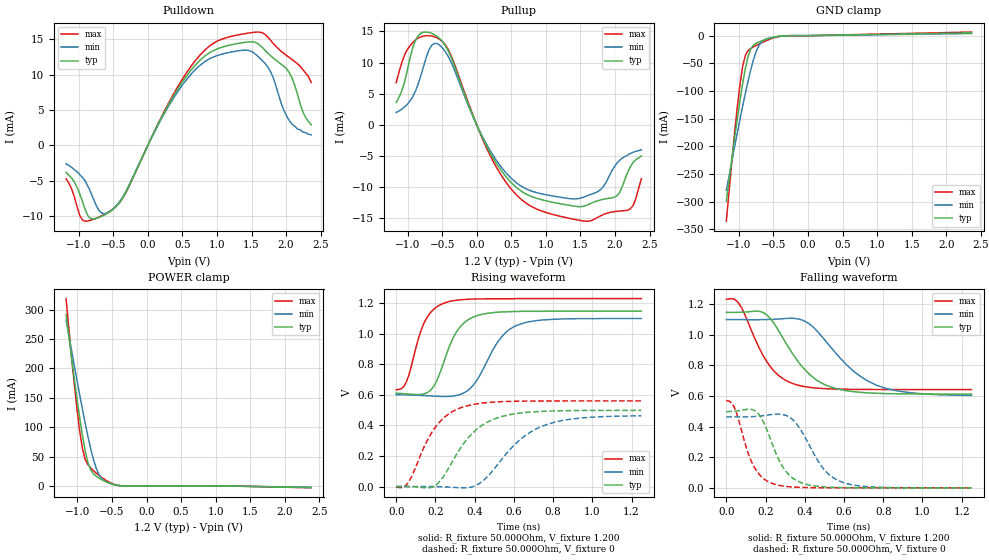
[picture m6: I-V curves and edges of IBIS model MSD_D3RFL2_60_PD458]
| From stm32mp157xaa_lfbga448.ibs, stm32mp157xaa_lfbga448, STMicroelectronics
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[Model] MSD_D3RFL2_60_PD458
Model_type   I/O
C_comp 2.402pF   2.316pF   2.526pF
Vinh = 820.000mV
Vinl = 380.000mV
Vmeas = 600.000mV
Vref = 600.000mV
[Model Spec]
Vinh   820.000mV   790.000mV   870.000mV
Vinl   380.000mV   350.000mV   430.000mV
Vmeas   600.000mV   570.000mV   650.000mV
Vref   600.000mV   570.000mV   650.000mV
[Temperature Range]   25.000   125.000   -40.000
[Voltage Range]   1.200V   1.140V   1.300V
[GND Clamp Reference]   0.00V   0.00V   0.00V
[Pulldown Reference]   0.00V   0.00V   0.00V
[POWER Clamp Reference]   1.200V   1.140V   1.300V
[Pullup Reference]   1.200V   1.140V   1.300V
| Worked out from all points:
|   slope of the pulldown table from 0 to 0.18 V, typ, clamps not added: 50.1 ohm
|   slope of the pullup table from 0 to 0.18 V, typ, clamps not added: 42.9 ohm
|   GND clamp passes 1 mA (typ) near -0.40 V on its own axis
|   POWER clamp passes 1 mA (typ) near -0.41 V on its own axis
|   rising waveform, R_fixture 50.000Ohm, V_fixture 1.200: 20-80 % time 108ps typ, 139ps min, 90.1ps max; typ from 0.61 V to 1.15 V
|   rising waveform, R_fixture 50.000Ohm, V_fixture 0: 20-80 % time 178ps typ, 220ps min, 148ps max; typ from 0.001 V to 0.498 V
|   falling waveform, R_fixture 50.000Ohm, V_fixture 1.200: 20-80 % time 185ps typ, 235ps min, 145ps max; typ from 1.15 V to 0.612 V
|   falling waveform, R_fixture 50.000Ohm, V_fixture 0: 20-80 % time 109ps typ, 136ps min, 92.8ps max; typ from 0.497 V to 0 V
[GND Clamp]
-1.182V   -299.1mA   -279.3mA   -335.3mA
-1.064V   -187mA     -201.5mA   -177mA
-984.9mV  -117.6mA   -151.3mA   -88.16mA
-945.5mV  -86.22mA   -127.1mA   -55.37mA
-906.1mV  -58.84mA   -103.8mA   -35.26mA
-866.7mV  -37.35mA   -81.5mA    -26.87mA
-787.9mV  -16.73mA   -42.8mA    -20.29mA
-709.1mV  -11.25mA   -17.38mA   -15.2mA
-630.3mV  -7.745mA   -7.438mA   -10.54mA
-512.1mV  -3.498mA   -2.984mA   -4.633mA
-315.1mV  -158.7uA   -224.9uA   -147.6uA
2.364V    4.99mA     3.837mA    6.535mA
[Power Clamp]
-1.164V   292mA      282.1mA    318.7mA
-1.085V   218.3mA    230.5mA    219.6mA
-1.006V   148.1mA    179.7mA    130.7mA
-966.7mV  115.5mA    154.8mA    92.95mA
-927.3mV  85.81mA    130.6mA    63.61mA
-887.9mV  60.1mA     107.1mA    45.52mA
-809.1mV  27.58mA    64.08mA    30.85mA
-730.3mV  16.84mA    30.96mA    22.19mA
-690.9mV  13.77mA    20.14mA    18.34mA
-572.7mV  6.533mA    6.447mA    8.649mA
-336.4mV  178.2uA    339.3uA    207.6uA
2.382V    -2.569mA   -2.119mA   -3.047mA
[Pulldown]
-1.182V   -3.8mA     -2.6mA     -4.7mA
-945.5mV  -7.91mA    -4.5mA     -10.51mA
-827.3mV  -10.3mA    -6.57mA    -10.56mA
-669.7mV  -10.01mA   -9.53mA    -9.94mA
-551.5mV  -9.372mA   -9.334mA   -9.3mA
-315.1mV  -6.567mA   -6.464mA   -6.607mA
551.5mV   9.677mA    9.197mA    10.13mA
906.1mV   13.16mA    12.3mA     14.13mA
1.261V    14.32mA    13.29mA    15.53mA
1.733V    13.06mA    11.13mA    15.34mA
2.009V    10.78mA    4.14mA     12.68mA
2.364V    2.9mA      1.5mA      8.9mA
[Pullup]
-1.164V   3.6mA      2.005mA    6.785mA
-1.045V   6.8mA      2.857mA    11.16mA
-887.9mV  13.51mA    5.344mA    13.62mA
-690.9mV  14.84mA    11.99mA    14.32mA
-454.5mV  12.73mA    11.77mA    12.85mA
175.8mV   -4.108mA   -3.772mA   -4.491mA
687.9mV   -10.95mA   -10.12mA   -12.35mA
1.476V    -13.14mA   -11.84mA   -15.31mA
1.791V    -12.06mA   -10.41mA   -14.62mA
1.988V    -11.63mA   -6.784mA   -13.94mA
2.224V    -6.7mA     -4.595mA   -13.49mA
2.382V    -5mA       -3.995mA   -8.654mA
[Ramp]
R_load=50.000Ohm
dV/dt_r   309.780mV/144.000ps  288.449mV/181.000ps  343.920mV/118.500ps
dV/dt_f   309.750mV/147.000ps  288.359mV/187.500ps  343.920mV/119.500ps
[Rising waveform]
R_fixture=50.000Ohm
V_fixture=1.200
V_fixture_min=1.140
V_fixture_max=1.300
0s        609.6mV    600.2mV    633.2mV
52ps      605.4mV    598.9mV    683.8mV
128ps     602.2mV    595.1mV    1.025V
166ps     619.9mV    592.6mV    1.121V
243ps     814.6mV    588.5mV    1.198V
294ps     980.1mV    592.2mV    1.215V
358ps     1.082V     621.8mV    1.223V
524ps     1.14V      956.2mV    1.227V
613ps     1.144V     1.052V     1.228V
1.25ns    1.146V     1.098V     1.228V
[Rising waveform]
R_fixture=50.000Ohm
V_fixture=0
0s        587.1uV    127.1uV    -3.676mV
64ps      191.8uV    470.4uV    31.75mV
192ps     960.1uV    245.9uV    374.1mV
332ps     259.6mV    -7.831mV   516.2mV
409ps     372.7mV    9.648mV    540mV
486ps     434mV      94.9mV     551.1mV
626ps     479.6mV    300.5mV    557.7mV
741ps     491.1mV    392.2mV    559.1mV
945ps     497.1mV    448.4mV    559.6mV
1.25ns    497.8mV    462.3mV    559.8mV
[Falling waveform]
R_fixture=50.000Ohm
V_fixture=1.200
V_fixture_min=1.140
V_fixture_max=1.300
0s        1.146V     1.098V     1.231V
64ps      1.146V     1.098V     1.203V
192ps     1.141V     1.098V     853.3mV
269ps     1.02V      1.102V     730.4mV
345ps     861.9mV    1.106V     678mV
422ps     742.3mV    1.071V     656.2mV
498ps     675.6mV    970.9mV    647.6mV
639ps     629.2mV    772.4mV    642.8mV
766ps     617mV      669.4mV    641.8mV
1.25ns    611.7mV    602.8mV    641.2mV
[Falling waveform]
R_fixture=50.000Ohm
V_fixture=0
0s        497.4mV    463.1mV    569.4mV
39ps      499.8mV    462.9mV    529.8mV
115ps     512.6mV    463.6mV    212.4mV
154ps     495.9mV    466.6mV    111mV
230ps     300.2mV    478mV      30.66mV
281ps     151.9mV    479.9mV    13.51mV
345ps     57.27mV    436mV      4.714mV
498ps     6.207mV    120.5mV    570.1uV
600ps     1.46mV     32.61mV    153.7uV
1.25ns    -731.6nV   -2.636uV   643.4nV
